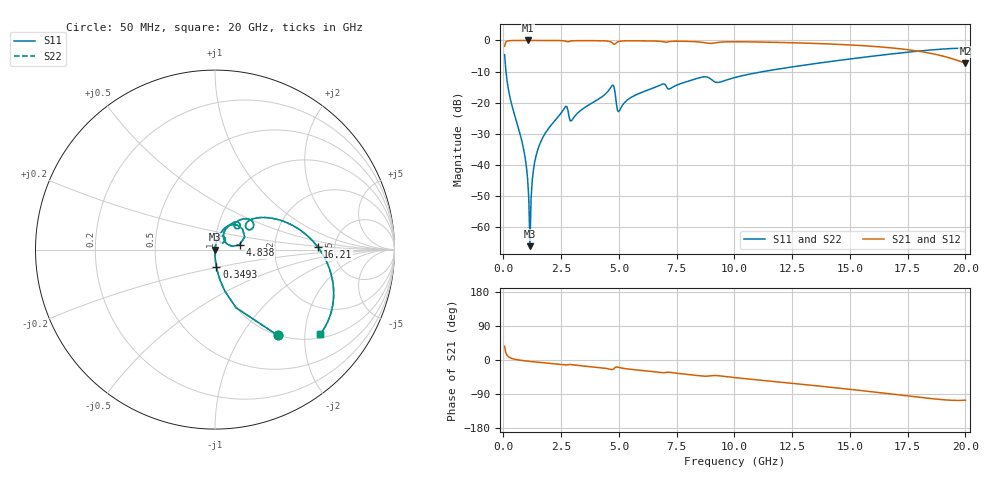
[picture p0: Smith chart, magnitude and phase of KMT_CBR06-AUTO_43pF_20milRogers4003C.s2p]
! Data measured by Modelithics Inc. support@modelithics.com 813-866-6335
! KEMET CBR06-AUTO 43pF, Pad Width= 0.851mm, Pad Length= 0.64mm, Pad Gap= 0.62mm, 20mil Rogers 4003C substrate Data, January 2022
# hz S ma R 50
! 2 Port Network Data from SP1.SP block
! freq  magS11  angS11  magS21  angS21  magS12  angS12  magS22  angS22
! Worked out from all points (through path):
!   401 points, 50 MHz to 20 GHz, reference 50 ohm
!   highest |S21| = 0.00 dB at 1.048 GHz (marker M1); lowest = -7.3 dB at 20 GHz (marker M2)
!   group delay of S21, straight-line fit = 15.6 ps
!   lowest |S11| = -66.2 dB at 1.147 GHz (marker M3), VSWR 1.00, Z = 50 + j0.00807 ohm
!   |S11| at or under -10 dB: 110.8 MHz to 11.26 GHz (11.15 GHz wide, 196 % of centre)
!   |S22| runs from -66.2 to -2.5 dB; largest |S21 - S12| = 0
!   S11 on the Smith chart (normalised r, x): 50 MHz: 1.00, -1.47; 349.2 MHz: 1.00, -0.19; 4.838 GHz: 1.32, +0.07; 16.21 GHz: 3.66, +0.17; 20 GHz: 1.11, -2.40
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5e7  0.5924 -53.8  0.8053 36.2  0.8053 36.2  0.5924 -53.8
3.4925e8  0.09538 -85.5  0.9951 4.3  0.9951 4.3  0.09538 -85.5
8.97875e8  0.01597 -90.5  0.9994 -2.0  0.9994 -2.0  0.01597 -90.5
9.97625e8  0.00903 -89.9  0.9995 -2.7  0.9995 -2.7  0.00903 -89.9
1.0475e9  0.005847 -88.6  0.9995 -3.0  0.9995 -3.0  0.005847 -88.6
1.14725e9  0.0004906 9.5  0.9995 -3.7  0.9995 -3.7  0.0004906 9.5
1.247e9  0.005616 80.5  0.9994 -4.3  0.9994 -4.3  0.005616 80.5
1.296875e9  0.008214 81.8  0.9994 -4.6  0.9994 -4.6  0.008214 81.8
1.396625e9  0.01321 82.4  0.9993 -5.3  0.9993 -5.3  0.01321 82.4
1.74575e9  0.02929 81.4  0.9988 -7.3  0.9988 -7.3  0.02929 81.4
2.6435e9  0.08203 66.4  0.9817 -13.1  0.9817 -13.1  0.08203 66.4
2.94275e9  0.05101 59.1  0.9824 -12.2  0.9824 -12.2  0.05101 59.1
3.391625e9  0.07727 72.1  0.9934 -15.3  0.9934 -15.3  0.07727 72.1
4.688375e9  0.1849 47.3  0.9285 -25.2  0.9285 -25.2  0.1849 47.3
4.838e9  0.14 10.9  0.8767 -19.6  0.8767 -19.6  0.14 10.9
5.0375e9  0.07586 49.2  0.9707 -20.2  0.9707 -20.2  0.07586 49.2
6.73325e9  0.187 54.7  0.9724 -32.3  0.9724 -32.3  0.187 54.7
1.0025e10  0.2537 40.3  0.953 -46.5  0.953 -46.5  0.2537 40.3
1.336662e10  0.4178 21.8  0.8983 -66.9  0.8983 -66.9  0.4178 21.8
1.62095e10  0.5716 1.6  0.7925 -85.6  0.7925 -85.6  0.5716 1.6
1.670825e10  0.6006 -2.5  0.7642 -89.1  0.7642 -89.1  0.6006 -2.5
2e10  0.752 -38.7  0.4296 -106.1  0.4296 -106.1  0.752 -38.7
